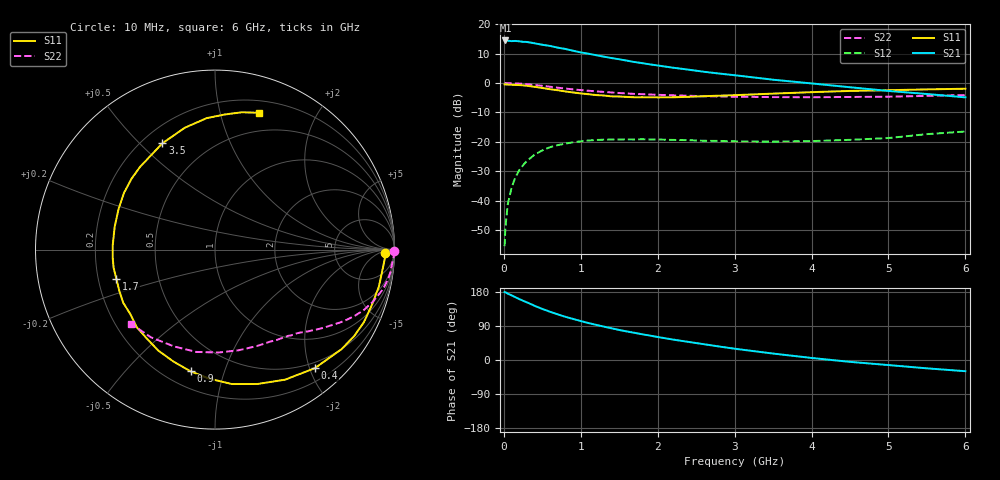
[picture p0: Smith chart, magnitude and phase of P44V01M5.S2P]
! SIEMENS Small Signal Semiconductors
! BFP182
! Si NPN RF Bipolar Junction Transistor in SOT143
! VCE = 4 V  IC = 1.5 mA
! Common Emitter S-Parameters:  March  1996
# GHz  S  MA  R  50
!  f  S11  S21  S12  S22
! GHz  MAG  ANG  MAG  ANG  MAG  ANG  MAG  ANG
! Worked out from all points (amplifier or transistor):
!   36 points, 10 MHz to 6 GHz, reference 50 ohm
!   highest |S21| = 14.5 dB at 20 MHz (marker M1)
!   |S21| within 3 dB of that: start of sweep to 819.3 MHz
!   unconditionally stable (mu >= 1): 2.422 GHz to end of sweep
!   at 250 MHz: K = 0.11, MSG = 21.0 dB, |S12| = -27.9 dB
!   at 1.4 GHz: K = 0.60, MSG = 13.8 dB, |S12| = -19.2 dB
!   at 6 GHz: K = 1.01, MAG = 5.1 dB, |S12| = -16.5 dB
!   S11 on the Smith chart (normalised r, x): 10 MHz: 32, -13; 400 MHz: 0.40, -2.09; 900 MHz: 0.30, -0.78; 1.7 GHz: 0.28, -0.14; 3.5 GHz: 0.28, +0.59; 6 GHz: 0.31, +1.32
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0.01  0.9476 -1.3  5.18 179.3  0.0017 84.5  0.9979 -0.5
0.02  0.9487 -2.5  5.279 178.7  0.0035 85.5  1 -1.0
0.05  0.9407 -6.4  5.23 175.2  0.0086 87.1  0.9956 -2.5
0.1  0.9361 -12.8  5.147 170.6  0.0167 80.9  0.9889 -4.9
0.15  0.9267 -19.7  5.18 165.7  0.0251 77.6  0.9858 -7.4
0.2  0.9231 -25.9  5.104 160.9  0.033 74.6  0.9777 -9.7
0.3  0.8971 -38.2  4.973 152.2  0.0478 67.1  0.9538 -14.3
0.4  0.8636 -49.9  4.729 143.0  0.0608 60.5  0.926 -18.3
0.5  0.8231 -61.7  4.461 134.7  0.0719 53.8  0.8965 -21.9
0.6  0.7852 -72.5  4.268 127.4  0.0814 48.3  0.8654 -25.0
0.7  0.7548 -82.9  3.987 120.5  0.0882 43.5  0.8333 -27.9
0.8  0.7191 -92.7  3.788 114.0  0.0936 39.2  0.8057 -30.3
0.9  0.6918 -101.3  3.532 108.4  0.0988 35.0  0.7803 -32.4
1.1  0.6453 -119.3  3.144 97.4  0.1058 28.2  0.7393 -36.3
1.4  0.5932 -142.6  2.653 83.7  0.1098 20.3  0.6915 -41.2
1.7  0.5731 -163.3  2.27 71.7  0.1104 15.0  0.653 -45.5
2.2  0.5732 167.3  1.819 53.9  0.1082 9.4  0.6183 -52.8
2.8  0.61 139.7  1.447 35.6  0.1041 6.9  0.591 -62.8
3.5  0.6609 116.3  1.139 17.0  0.1013 8.4  0.5763 -76.6
4.5  0.734 93.6  0.848 -4.9  0.1085 13.7  0.5796 -100.4
5.5  0.7796 78.9  0.651 -22.0  0.1356 17.6  0.605 -126.1
6  0.8002 72.3  0.571 -29.6  0.1503 15.3  0.6253 -138.8
